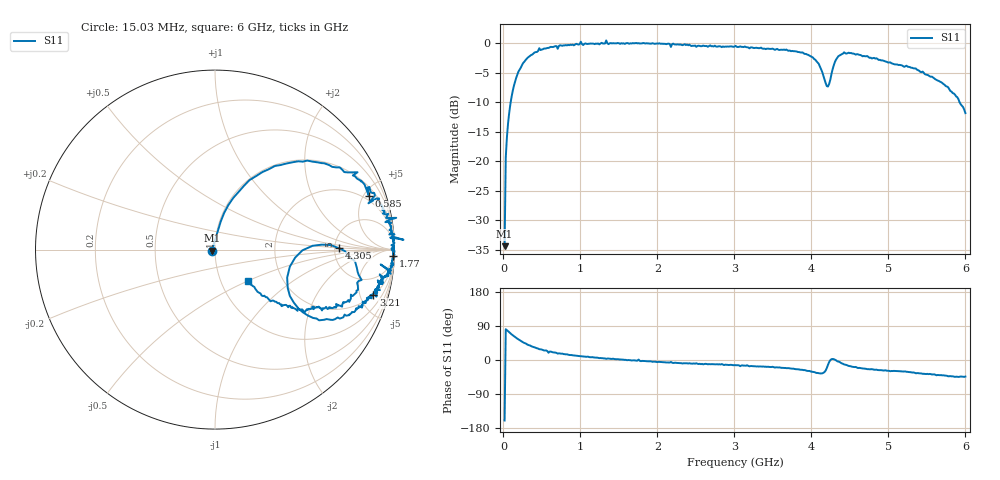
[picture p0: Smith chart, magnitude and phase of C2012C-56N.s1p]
!	Network	Analyzer	HP8753E.07.74:	Oct	30	2002	Serial	No.	JP38451487
!	Hewlett-Packard
!	7	Sep	2009	10:57:03
!	Frequency	S11
#	HZ	S	RI	R	50
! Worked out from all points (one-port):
!   400 points, 15.03 MHz to 6 GHz, reference 50 ohm
!   lowest |S11| = -34.4 dB at 15.03 MHz (marker M1), VSWR 1.04, Z = 48.2 - j0.636 ohm
!   |S11| at or under -10 dB: start of sweep to 94.34 MHz; 5.923 GHz to end of sweep
!   S11 on the Smith chart (normalised r, x): 15.03 MHz: 0.96, -0.01; 585 MHz: 1.61, +5.47; 1.77 GHz: 13, -53; 3.21 GHz: 2.01, -6.51; 4.305 GHz: 5.45, +0.16; 6 GHz: 1.34, -0.51
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1.502992e7  -0.0178 -0.00659
3.002985e7  0.0164 0.106
6.00297e7  0.0503 0.203
1.200294e8  0.162 0.356
2.850286e8  0.514 0.496
4.650277e8  0.794 0.431
5.850271e8  0.858 0.298
7.650262e8  0.907 0.275
1.005025e9  1.01 0.177
1.245024e9  0.971 0.0838
1.335023e9  1.05 0.0549
1.365023e9  0.976 0.067
1.515022e9  0.983 0.0245
1.770021e9  0.991 -0.0353
2.265019e9  0.966 -0.133
3.015015e9  0.919 -0.226
3.210014e9  0.883 -0.253
3.765011e9  0.787 -0.33
4.06501e9  0.58 -0.394
4.140009e9  0.465 -0.328
4.200009e9  0.402 -0.156
4.260009e9  0.544 0.0214
4.305008e9  0.69 0.00772
4.425008e9  0.817 -0.169
4.515007e9  0.789 -0.238
5.265004e9  0.534 -0.331
5.775001e9  0.309 -0.288
6e9  0.184 -0.176
